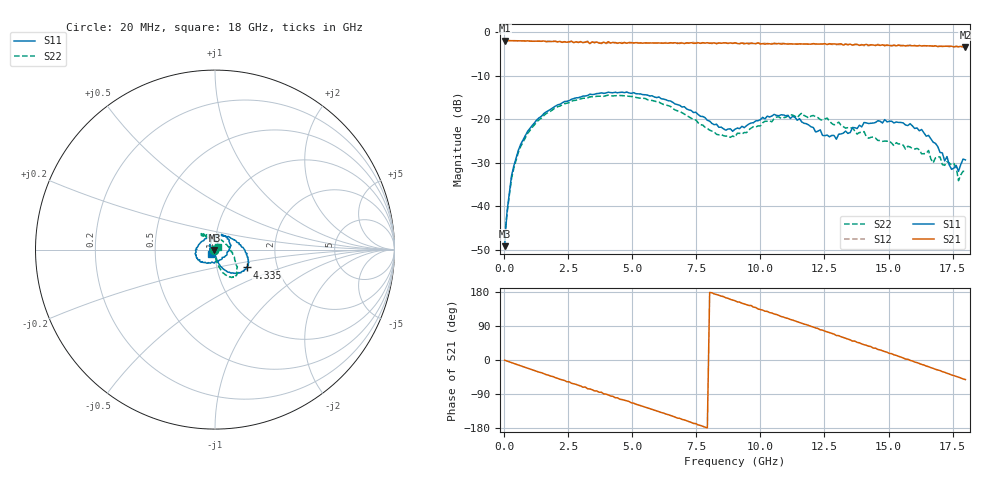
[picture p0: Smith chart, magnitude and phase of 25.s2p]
!Agilent Technologies,N5230A,US43500223,A.07.50.48
!Agilent N5230A: A.07.50.48
!Date: Tuesday, February 02, 2016 10:21:14
!Correction: S11(Full 2 Port(1,2))
!S21(Full 2 Port(1,2))
!S12(Full 2 Port(1,2))
!S22(Full 2 Port(1,2))
!S2P File: Measurements: S11, S21, S12, S22:
# Hz S  RI  R 50
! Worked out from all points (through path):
!   201 points, 20 MHz to 18 GHz, reference 50 ohm
!   highest |S21| = -1.94 dB at 20 MHz (marker M1); lowest = -3.4 dB at 18 GHz (marker M2)
!   group delay of S21, straight-line fit = 63.2 ps
!   lowest |S11| = -49.2 dB at 20 MHz (marker M3), VSWR 1.01, Z = 49.7 - j0.174 ohm
!   |S11| at or under -10 dB: start of sweep to end of sweep
!   |S22| runs from -46.8 to -14.5 dB; largest |S21 - S12| = 0.033
!   S11 on the Smith chart (normalised r, x): 20 MHz: 0.99, -0.00; 4.335 GHz: 1.40, -0.29; 18 GHz: 0.95, -0.05
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2e7  -0.00301 -0.00175  0.7995 -0.0071  0.8021 -0.00918  -0.00446 -0.000988
1.099e8  -0.00328 -0.00773  0.798 -0.0375  0.7998 -0.0381  -0.00386 -0.007
2.897e8  -0.000207 -0.0224  0.7908 -0.0969  0.7908 -0.0977  -0.000689 -0.0208
8.291e8  0.0135 -0.0639  0.7452 -0.2652  0.7453 -0.2667  0.00822 -0.0607
1.6382e9  0.0497 -0.1106  0.6081 -0.4838  0.61 -0.4861  0.0312 -0.1115
3.0766e9  0.13 -0.1303  0.237 -0.7188  0.2431 -0.7267  0.0832 -0.153
4.3352e9  0.1782 -0.0992  -0.1239 -0.744  -0.114 -0.7535  0.1139 -0.1467
6.0433e9  0.1785 -0.0222  -0.5431 -0.518  -0.5463 -0.5161  0.1247 -0.0957
7.5716e9  0.0965 0.0593  -0.7456 -0.1147  -0.7636 -0.1135  0.0901 -0.0119
9.01e9  -0.0333 0.0692  -0.6927 0.3019  -0.6851 0.3001  0.023 0.0581
1.05383e10  -0.1111 -0.0235  -0.3872 0.6361  -0.3812 0.6267  -0.0563 0.0852
1.20666e10  -0.0261 -0.0758  0.0393 0.737  0.0551 0.7291  -0.069 0.0861
1.29656e10  0.0398 -0.0435  0.3113 0.6564  0.3048 0.648  -0.0482 0.0743
1.40444e10  0.0893 0.0205  0.542 0.4594  0.5338 0.4498  -0.0248 0.0677
1.50333e10  0.0613 0.0721  0.67 0.2075  0.6773 0.1971  -0.00597 0.0558
1.62919e10  -0.00592 0.0759  0.6777 -0.1395  0.6791 -0.1572  0.014 0.0374
1.71909e10  -0.0269 0.0195  0.581 -0.3685  0.5646 -0.382  0.0164 0.0245
1.72808e10  -0.0299 0.0221  0.5647 -0.3951  0.554 -0.4129  0.0262 0.0192
1.74606e10  -0.0265 0.00209  0.5319 -0.4384  0.5202 -0.456  0.0219 0.0205
1.76404e10  -0.029 -0.00548  0.5009 -0.4722  0.4853 -0.479  0.0215 0.0177
1.77303e10  -0.0248 -0.00441  0.4779 -0.4825  0.454 -0.5041  0.0176 0.00875
1.8e10  -0.0229 -0.0253  0.419 -0.5289  0.3962 -0.5355  0.0187 0.0167
